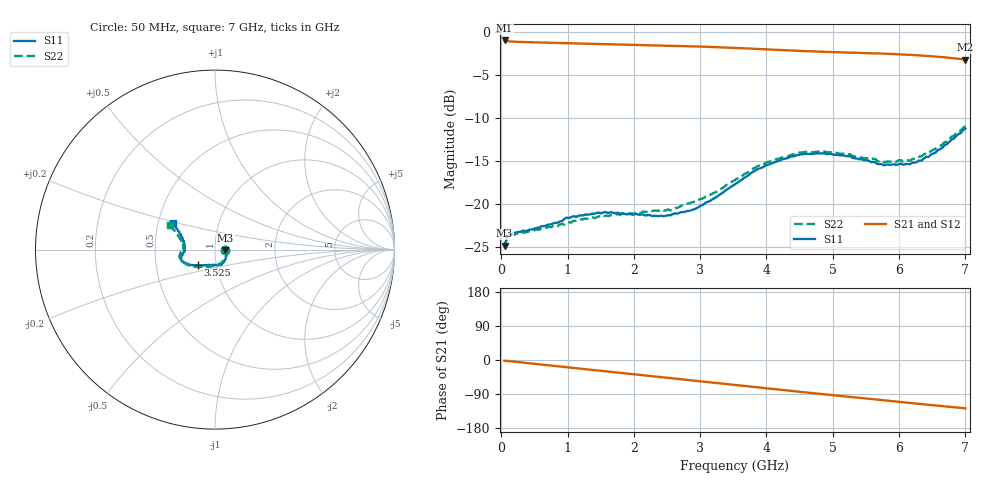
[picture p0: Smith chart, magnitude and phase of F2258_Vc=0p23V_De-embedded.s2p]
! Integrated Device Technology
! Corporate Headquarters
! 6024 Silver Creek Valley Road
! San Jose, CA 95138  USA
! Phone:  1-408-284-8200
! Toll Free:  1-800-223-1366
! Webpage:  http://www.idt.com/
! Timing and RF Division
! 515 Groton Road, Suite 102
! Westford, MA 01886-6024
! Device:  F2258
! Description: Voltage Variable RF Attenuator
! Frequency:  50.0 -  6000.00 MHz
! Package:  3x3 mm Thin QFN Plastic Package: 16 pin
! Ports:  2 RF, 2 DC
!  Pin  1  = NC
!  Pin  2  = NC
!  Pin  3  = RF2  = Port 2
!  Pin  4  = GND
!  Pin  5  = Vdd
!  Pin  6  = NC
!  Pin  7  = VCTRL
!  Pin  8  = NC
!  Pin  9  = GND
!  Pin 10  = RF1  = Port 1
!  Pin 11  = NC
!  Pin 12  = NC
!  Pin 13  = NC
!  Pin 14  = NC
!  Pin 15  = NC
!  Pin 16  = NC
! Vcntrl:  0.230 Volts
! Vdd:  +3.300 Volts
! Current:  1.079 mA
! Data:  The device was measured on a the F2258 evaluation board which has
!  individual transmission lines to the RF pins.  Data was collected
!  using a calibrated network analyzer.  The evaluation board was
!  de-embedded using a TRL calibration technique.
!  The reference plane is the edge of the package pin.
! Misc:  SN 10
!  Action Tracker AT0285
! Date Measured:  2014-12-10
! Date:  2016-01-13  MJV
! Note:
!  Integrated Device Technology supplies this data as a sample of measured
!  data at the package pin for this product.  Your particular data for this
!  product may vary.
!  Data was taken at 25 degrees C.
!  Integrated Device Technology reserves the right to change this data at anytime.
!Freq_(GHz)  S11M_(dB)  S11P_(deg)  S21M_(dB)  S21P_(deg)  S12M_(dB)  S12P_(deg)  S22M_(dB)  S22P_(deg)
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# GHz S dB R 50
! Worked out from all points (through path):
!   201 points, 50 MHz to 7 GHz, reference 50 ohm
!   highest |S21| = -0.96 dB at 50 MHz (marker M1); lowest = -3.2 dB at 7 GHz (marker M2)
!   group delay of S21, straight-line fit = 50.5 ps
!   lowest |S11| = -24.8 dB at 50 MHz (marker M3), VSWR 1.12, Z = 56.1 - j0.391 ohm
!   |S11| at or under -10 dB: start of sweep to end of sweep
!   |S22| runs from -24.9 to -10.9 dB; largest |S21 - S12| = 0.00039
!   S11 on the Smith chart (normalised r, x): 50 MHz: 1.12, -0.01; 3.525 GHz: 0.81, -0.15; 7 GHz: 0.60, +0.19
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0.05  -24.84 -3.5  -0.96 -1.9  -0.96 -1.9  -24.89 -3.1
0.08475  -23.87 -5.9  -1.03 -2.4  -1.03 -2.4  -23.94 -5.5
0.15425  -23.38 -9.2  -1.09 -3.6  -1.09 -3.6  -23.56 -9.4
0.71025  -22.36 -37.1  -1.22 -14.1  -1.22 -14.1  -22.66 -38.6
0.91875  -21.97 -46.8  -1.26 -18.0  -1.26 -18.0  -22.30 -50.3
0.98825  -21.58 -50.9  -1.27 -19.3  -1.27 -19.3  -22.16 -54.7
1.2315  -21.33 -59.2  -1.33 -23.8  -1.33 -23.8  -21.77 -63.6
1.6485  -20.93 -70.9  -1.41 -31.4  -1.41 -31.4  -21.29 -76.7
2.37825  -21.40 -92.3  -1.54 -44.8  -1.54 -44.8  -20.76 -94.2
2.552  -21.30 -98.2  -1.57 -48.0  -1.57 -48.0  -20.72 -99.6
2.93425  -20.53 -114.9  -1.65 -55.1  -1.65 -55.1  -19.71 -112.9
3.525  -17.70 -137.7  -1.82 -66.2  -1.82 -66.2  -17.20 -135.6
4.0115  -15.43 -151.3  -2.00 -75.2  -2.00 -75.2  -15.11 -151.0
4.46325  -14.28 -159.7  -2.16 -83.4  -2.16 -83.4  -14.06 -162.0
4.7065  -14.15 -163.0  -2.23 -87.7  -2.23 -87.7  -13.96 -166.3
5.2625  -14.43 -169.9  -2.38 -97.4  -2.39 -97.4  -14.20 -174.3
5.6795  -15.35 -176.7  -2.47 -104.6  -2.47 -104.6  -15.02 -179.7
5.85325  -15.42 179.1  -2.52 -107.8  -2.53 -107.8  -15.05 175.7
6.166  -15.35 171.3  -2.63 -113.4  -2.63 -113.4  -14.96 169.8
6.33975  -14.93 165.0  -2.71 -116.5  -2.71 -116.5  -14.42 165.4
6.722  -13.02 153.3  -2.95 -123.1  -2.95 -123.1  -12.71 156.4
7  -11.20 147.9  -3.19 -127.4  -3.19 -127.4  -10.91 151.4
